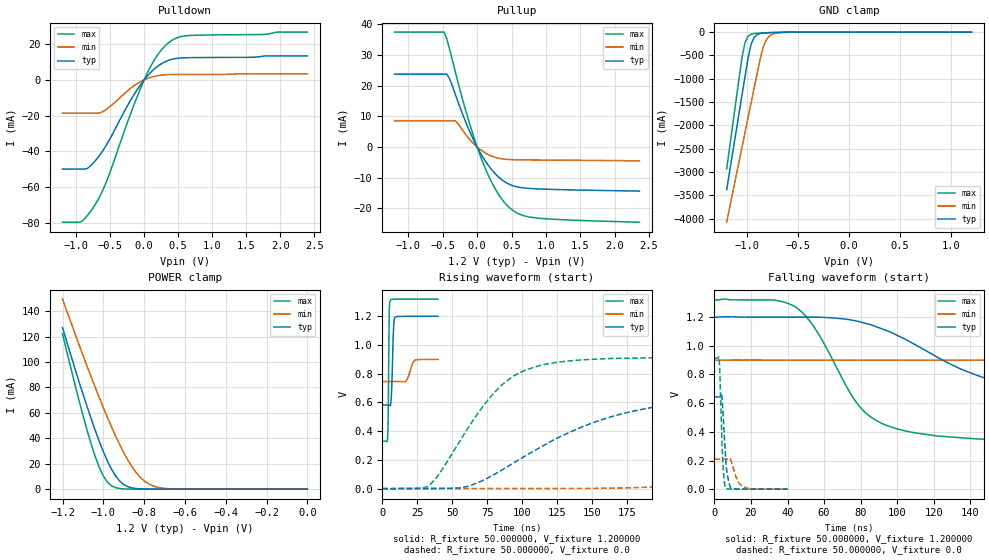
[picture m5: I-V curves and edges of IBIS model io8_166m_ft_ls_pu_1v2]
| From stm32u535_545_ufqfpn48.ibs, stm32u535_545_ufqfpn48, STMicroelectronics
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|   Model io8_166m_ft_ls_pu_1v2
[Model]  io8_166m_ft_ls_pu_1v2
Model_type I/O
Polarity   Non-Inverting
Enable   Active-Low
Vinl =   0.360000V
Vinh =   0.840000V
Vmeas =  0.600000V
Cref =   50.000000pF
Rref =   100.000000M
Vref =   0.0V
C_comp   3.151400pF   3.086700pF   3.197700pF
[Temperature Range]   25.000000   0.140000k   -40.000000
[Pullup Reference]   1.200000V   0.900000V   1.320000V
[Pulldown Reference]   0.0V   0.0V   0.0V
[POWER Clamp Reference]   1.200000V   0.900000V   1.320000V
[GND Clamp Reference]   0.0V   0.0V   0.0V
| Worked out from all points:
|   slope of the pulldown table from 0 to 0.18 V, typ, clamps not added: 25.4 ohm
|   slope of the pullup table from 0 to 0.18 V, typ, clamps not added: 27.8 ohm
|   GND clamp passes 1 mA (typ) near -0.51 V on its own axis
|   POWER clamp passes 1 mA (typ) near -0.86 V on its own axis
|   rising waveform, R_fixture 50.000000, V_fixture 1.200000: 20-80 % time 1.12ns typ, 3.03ns min, 550ps max; typ from 0.583 V to 1.2 V
|   rising waveform, R_fixture 50.000000, V_fixture 0.0: 20-80 % time 83.8ns typ, 204ns min, 40.6ns max; typ from 0 V to 0.643 V
|   falling waveform, R_fixture 50.000000, V_fixture 1.200000: 20-80 % time 70.8ns typ, 188ns min, 28.2ns max; typ from 1.2 V to 0.583 V
|   falling waveform, R_fixture 50.000000, V_fixture 0.0: 20-80 % time 1.99ns typ, 3.69ns min, 1.49ns max; typ from 0.643 V to 0 V
[Pulldown]
|Voltage   I(typ)   I(min)   I(max)
-1.2V     -49.86mA   -18.57mA   -79.56mA
-920mV    -49.86mA   -18.57mA   -79.19mA
-840mV    -49.6mA    -18.57mA   -76.08mA
-720mV    -45.32mA   -18.57mA   -69.74mA
-560mV    -36.71mA   -16.58mA   -57.44mA
-200mV    -11.43mA   -4.74mA    -19.03mA
0V        0A         0A         0A
160mV     6.477mA    2.075mA    11.78mA
360mV     10.99mA    2.989mA    20.81mA
480mV     12.07mA    3.054mA    23.52mA
640mV     12.43mA    3.074mA    24.76mA
2.4V      13.45mA    3.36mA     26.76mA
[Pullup]
|Voltage   I(typ)   I(min)   I(max)
-1.2V     23.71mA    8.575mA    37.42mA
-480mV    23.71mA    8.575mA    37.42mA
-440mV    23.71mA    8.575mA    35.14mA
-400mV    22.24mA    8.575mA    31.81mA
-320mV    17.36mA    8.575mA    24.69mA
-120mV    5.681mA    2.787mA    8.394mA
80mV      -3.179mA   -1.366mA   -4.88mA
280mV     -9.096mA   -3.479mA   -14.29mA
520mV     -12.61mA   -4.111mA   -20.65mA
680mV     -13.33mA   -4.182mA   -22.38mA
920mV     -13.66mA   -4.239mA   -23.22mA
2.36V     -14.4mA    -4.5mA     -24.47mA
[GND_clamp]
|Voltage   I(typ)   I(min)   I(max)
-1.2V     -3.379A    -4.076A    -2.932A
-1.05V    -1.35A     -2.47A     -550.7mA
-1.02V    -947.8mA   -2.149A    -221.5mA
-990mV    -552.4mA   -1.829A    -88.44mA
-960mV    -255.3mA   -1.51A     -44.87mA
-930mV    -111.8mA   -1.191A    -30.68mA
-870mV    -28.36mA   -564.6mA   -21.34mA
-840mV    -18.65mA   -309.5mA   -18.49mA
-810mV    -14.07mA   -161.6mA   -15.92mA
-780mV    -11.37mA   -83.33mA   -13.53mA
-600mV    -3.009mA   -4.322mA   -3.091mA
1.2V      0A         13.65nA    0A
[POWER_clamp]
|Voltage   I(typ)   I(min)   I(max)
-1.2V     127mA      149.4mA    122.2mA
-1.12V    84.98mA    114mA      70.29mA
-1.06V    55.52mA    88.42mA    35.69mA
-1.02V    37.64mA    72.04mA    17.19mA
-1V       29.52mA    64.13mA    10.33mA
-960mV    15.7mA     48.99mA    2.596mA
-900mV    3.636mA    28.77mA    207.8uA
-840mV    502.9uA    13.24mA    43.45uA
-800mV    129uA      6.535mA    43.45uA
-740mV    26.2uA     1.726mA    43.45uA
-620mV    25.1uA     82.33uA    35.72uA
0V        0A         17.36nA    0A
[Ramp]
| variable   typ   min   max
dV/dt_r  0.38566/83.69603n   0.12535/0.20373u   0.54818/40.55762n
dV/dt_f  0.37043/70.74310n   92.08800m/0.18810u  0.59405/28.06343n
R_load = 50.000000
[Rising Waveform]
R_fixture= 50.000000
V_fixture= 1.200000
V_fixture_min= 0.900000
V_fixture_max= 1.320000
|time   V(typ)   V(min)   V(max)
0s        582.6mV    746.1mV    329.9mV
3.764ns   582.7mV    746.1mV    361.4mV
4.244ns   582.7mV    746.1mV    541mV
4.885ns   581.2mV    746.1mV    1.195V
5.606ns   578mV      746.1mV    1.309V
6.567ns   671.7mV    746.1mV    1.318V
8.008ns   1.115V     746.1mV    1.319V
8.889ns   1.19V      746.1mV    1.319V
22.82ns   1.2V       891.3mV    1.32V
39.88ns   1.2V       900mV      1.32V
[Rising Waveform]
R_fixture= 50.000000
V_fixture= 0.0
V_fixture_min= 0.0
V_fixture_max= 0.0
|time   V(typ)   V(min)   V(max)
0s        434.2uV    495.9uV    378.8uV
34.03ns   1.423mV    890.3uV    26.88mV
60.06ns   13.38mV    895.1uV    402.7mV
86.09ns   132.9mV    957.4uV    726.4mV
102.1ns   226.9mV    1.02mV     824.5mV
134.1ns   392.7mV    1.506mV    889.7mV
192.2ns   563.5mV    10.93mV    910.9mV
274.3ns   629.6mV    62.99mV    914mV
516.5ns   643.1mV    185.8mV    914mV
997ns     643.3mV    209.9mV    914mV
[Falling Waveform]
R_fixture= 50.000000
V_fixture= 1.200000
V_fixture_min= 0.900000
V_fixture_max= 1.320000
|time   V(typ)   V(min)   V(max)
0s        1.2V       900mV      1.32V
44.04ns   1.2V       900mV      1.273V
54.05ns   1.2V       900mV      1.14V
82.08ns   1.158V     900mV      539.4mV
98.1ns    1.084V     900mV      427.5mV
124.1ns   904.9mV    900mV      369mV
170.2ns   706.1mV    898.7mV    339.3mV
252.3ns   610.1mV    878.8mV    330.7mV
494.5ns   582.7mV    768.3mV    329.9mV
997ns     582.6mV    746.1mV    329.9mV
[Falling Waveform]
R_fixture= 50.000000
V_fixture= 0.0
V_fixture_min= 0.0
V_fixture_max= 0.0
|time   V(typ)   V(min)   V(max)
0s        643.3mV    209.9mV    914mV
2.563ns   643.2mV    210mV      910mV
3.924ns   656.9mV    210mV      410.1mV
4.404ns   591.9mV    210mV      235mV
6.006ns   239.2mV    209.6mV    11.06mV
6.967ns   109.1mV    211.7mV    3.385mV
9.049ns   6.453mV    199.2mV    944.9uV
12.89ns   860uV      54.58mV    527.3uV
16.9ns    458.7uV    12.01mV    526.9uV
39.88ns   434.2uV    495.9uV    378.8uV
